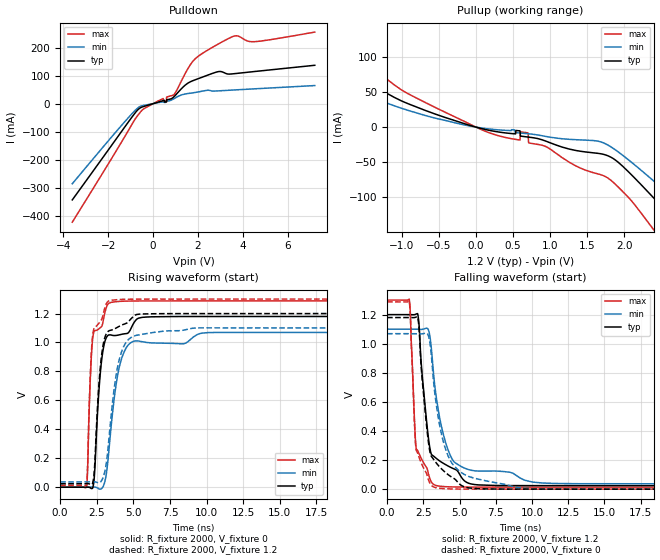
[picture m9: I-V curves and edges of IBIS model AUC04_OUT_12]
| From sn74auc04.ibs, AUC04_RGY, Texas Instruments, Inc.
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[Model]   AUC04_OUT_12
Model_type  Output
Vref =   0
Rref =   2000
Cref =   15p
Vmeas =   0.6
| variable   typ   min   max
C_comp   3.5pF   NA   NA
| C_pullup   6.25pF   0.87pF   16.76pF
| C_pulldown   6.74pF   4.64pF   15.17pF
[Temperature Range]   40   100   -40
| Ambient temperature   25   85   -40
[Voltage range]   1.2   1.1   1.3
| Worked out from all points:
|   slope of the pulldown table from 0 to 0.18 V, typ, clamps not added: 41.6 ohm
|   slope of the pullup table from 0 to 0.18 V, typ, clamps not added: 38.4 ohm
|   rising waveform, R_fixture 2000, V_fixture 0: 20-80 % time 504ps typ, 809ps min, 313ps max; typ from 0 V to 1.18 V
|   falling waveform, R_fixture 2000, V_fixture 1.2: 20-80 % time 705ps typ, 1.16ns min, 404ps max; typ from 1.2 V to 0.024 V
|   rising waveform, R_fixture 2000, V_fixture 1.2: 20-80 % time 494ps typ, 802ps min, 304ps max; typ from 0.024 V to 1.2 V
|   falling waveform, R_fixture 2000, V_fixture 0: 20-80 % time 717ps typ, 1.17ns min, 406ps max; typ from 1.18 V to 0 V
[Pulldown]
| AUC04_OUT_12
|   Voltage   I(typ)   I(min)   I(max)
-3.6V     -343.7mA   -285.9mA   -423.2mA
-650mV    -19.7mA    -13.52mA   -38.65mA
-370mV    -8.898mA   -5.454mA   -16.13mA
590mV     6.193mA    8.414mA    8.677mA
605mV     13.32mA    8.578mA    23.51mA
930mV     24.77mA    17.77mA    32.46mA
1.61V     76.08mA    36.87mA    132.9mA
1.985V    88.47mA    41.53mA    167.6mA
2.92V     114.6mA    45.74mA    213.7mA
3.635V    107.2mA    49.01mA    241.8mA
4.51V     114.7mA    52.9mA     221.3mA
7.2V      137mA      64.62mA    255.5mA
[Pullup]
| AUC04_OUT_12
|   Voltage   I(typ)   I(min)   I(max)
-3.6V     236.7mA    114.8mA    301.3mA
-2.45V    144.6mA    76.08mA    187.3mA
-2.055V   110.8mA    79.63mA    148.3mA
-675mV    23.63mA    16.44mA    34.85mA
270mV     -6.37mA    -3.622mA   -11.25mA
700mV     -14.19mA   -9.421mA   -8.122mA
715mV     -14.38mA   -9.579mA   -22.55mA
1.785V    -41.24mA   -25.95mA   -73.29mA
2.43V     -105mA     -79.97mA   -151.5mA
2.8V      -147.1mA   -114.5mA   -203.3mA
3.29V     -203.3mA   -161.3mA   -270.8mA
7.2V      -648.3mA   -542.2mA   -796.5mA
[Ramp]
| AUC04_OUT_12
| variable   typ   min   max
dV/dt_r   0.71/5.07E-10   0.65/8.18E-10   0.78/3.19E-10
dV/dt_f   0.71/7.13E-10   0.64/1.16E-09   0.78/4.03E-10
R_load = 2000
[Rising Waveform]
| AUC04_OUT_12
R_fixture =   2000
C_fixture =   0
L_fixture =   0
V_fixture =   0
V_fixture_min = 0
V_fixture_max = 0
|   Time   V(typ)   V(min)   V(max)
0s        8.805nV    38.15nV    771.5pV
1.82ns    657.1uV    388.2uV    2.742mV
2.04ns    -2.914mV   772.8uV    702.2mV
2.225ns   -3.635mV   1.216mV    1.03V
2.34ns    80.82mV    1.257mV    1.08V
2.795ns   843.3mV    -11.32mV   1.107V
3.33ns    1.052V     256mV      1.271V
4.01ns    1.052V     817.4mV    1.284V
4.955ns   1.122V     1.006V     1.286V
23.3ns    1.18V      1.069V     1.287V
[Falling Waveform]
| AUC04_OUT_12
R_fixture =   2000
C_fixture =   0
L_fixture =   0
V_fixture =   1.2
V_fixture_min = 1.1
V_fixture_max = 1.3
|   Time   V(typ)   V(min)   V(max)
0s        1.2V       1.1V       1.3V
1.53ns    1.2V       1.1V       1.307V
1.6ns     1.2V       1.1V       1.229V
1.955ns   1.201V     1.1V       348.3mV
2.115ns   1.206V     1.099V     264.2mV
2.865ns   344.7mV    1.093V     101.8mV
3.235ns   225.3mV    768.3mV    31.64mV
4.185ns   160.7mV    276.5mV    16.44mV
5.485ns   47.18mV    139.4mV    14.41mV
23.3ns    24.06mV    36.69mV    13.89mV
[Rising Waveform]
| AUC04_OUT_12
R_fixture =   2000
C_fixture =   0
L_fixture =   0
V_fixture =   1.2
V_fixture_min = 1.1
V_fixture_max = 1.3
|   Time   V(typ)   V(min)   V(max)
0s        23.98mV    36.61mV    13.86mV
1.82ns    24.56mV    36.95mV    21.04mV
2.035ns   21.67mV    37.24mV    715.3mV
2.21ns    25.37mV    37.52mV    1.041V
2.335ns   117.4mV    37.52mV    1.101V
2.785ns   872.3mV    39.31mV    1.15V
3.305ns   1.079V     307.2mV    1.286V
4ns       1.11V      868.1mV    1.297V
5.015ns   1.181V     1.044V     1.299V
23.3ns    1.2V       1.1V       1.3V
[Falling Waveform]
| AUC04_OUT_12
R_fixture =   2000
C_fixture =   0
L_fixture =   0
V_fixture =   0
V_fixture_min = 0
V_fixture_max = 0
|   Time   V(typ)   V(min)   V(max)
0s        1.18V      1.069V     1.287V
1.53ns    1.18V      1.069V     1.293V
1.945ns   1.181V     1.069V     346.7mV
2.115ns   1.183V     1.068V     245.4mV
2.855ns   323.7mV    1.056V     66.07mV
3.19ns    207.9mV    763.2mV    16.5mV
3.59ns    157.3mV    460.8mV    6.419mV
4.095ns   109.3mV    259.2mV    2.668mV
5.63ns    8.582mV    87.45mV    459.4uV
23.3ns    81.19uV    59.77uV    31.08uV
